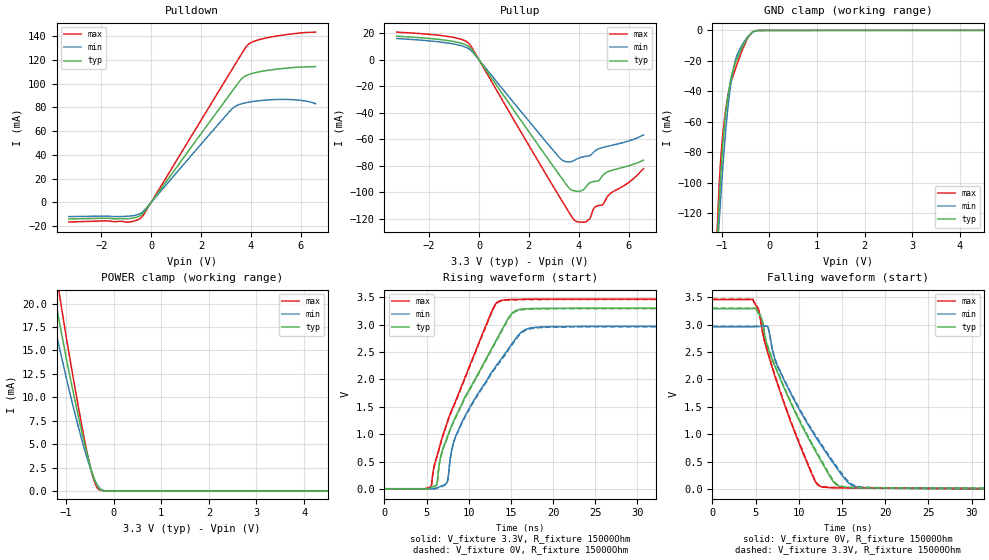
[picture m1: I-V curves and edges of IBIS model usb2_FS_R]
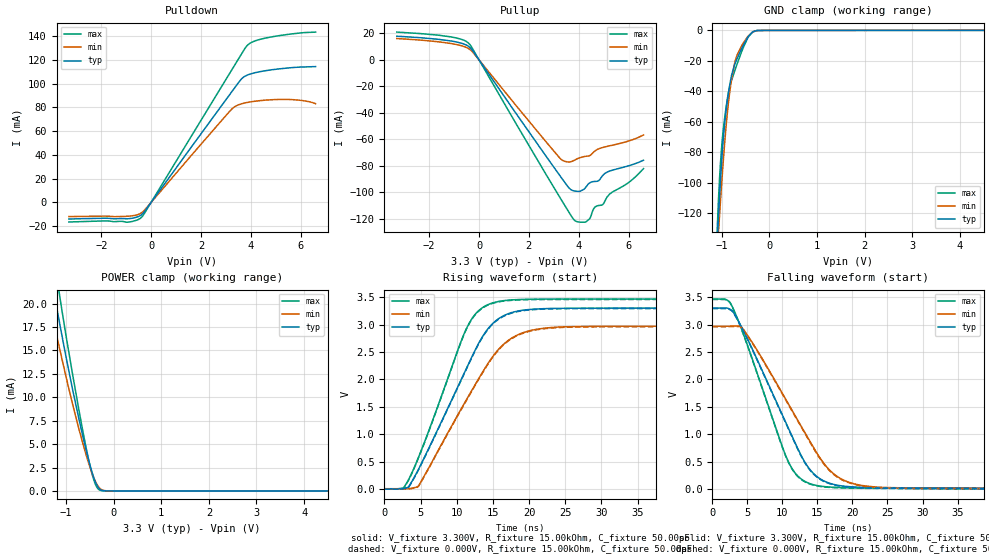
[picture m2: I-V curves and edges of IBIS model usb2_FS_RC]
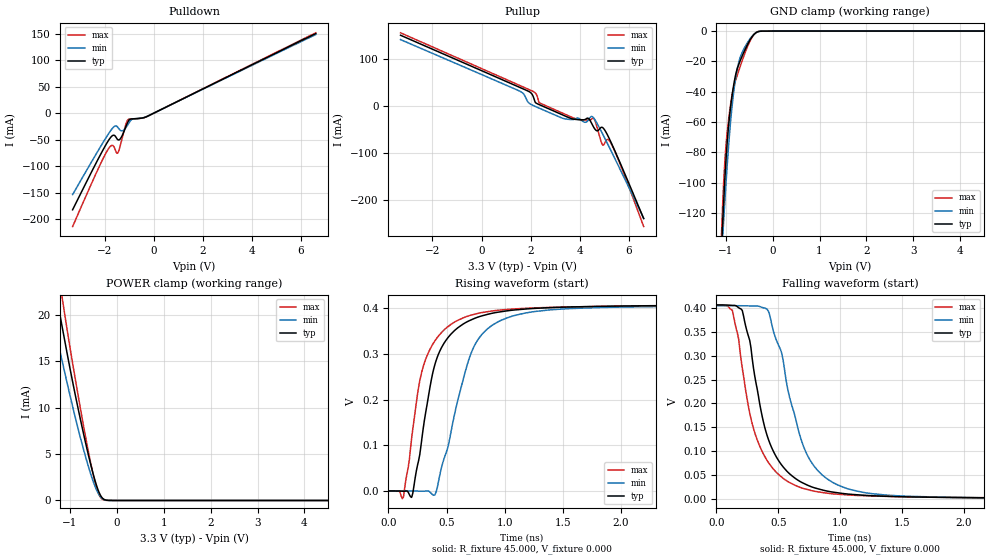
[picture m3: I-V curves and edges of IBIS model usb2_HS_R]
| Texas Instruments Incorporated
| Four-Port USB 2.0 Hub
| Marketing part#   Voltage Range   Package-type   Temperature
| TUSB4041PAP   2.97V - 3.465V   64-Pin PAP   -40 to 85 C
[IBIS Ver]   4.1
[File name]   tusb4041IPAP.ibs
[File Rev]   1.0
[Date]   05/22/2014
[Source]   Model built from TISPICE simulations at:
   Texas Instruments Incorporated.
   Analog-eLab, HPA
   12500 TI Blvd
   Dallas, TX -75243
[Notes]   Rev 1.0: 09/08/2017
   - Model based on v1.0 IBIS model for TUSB8041q1 dated 02/28/2014
[Disclaimer] This product is designed as an aid for customers of Texas Instruments.
   No warranties, either expressed or implied, with respect to this third
   party software (if any) or with respect to its fitness for any
   particular purpose is claimed by Texas Instruments or the author. The
   software (if any) is provided solely on an "as is" basis. The entire
   risk as to its quality and performance is with the customer
[Copyright]   (C)Copyright 2014 Texas Instruments Incorporated.
   All rights reserved.
|   TUSB8041
[Component]   TUSB4041
[Manufacturer]  Texas Instruments Incorporated
[Package]   |64-pin PAP
|   typ   min   max
R_pkg   0.2389   0.0142   0.3346
L_pkg   2.3741nH   1.4298nH   2.8522nH
C_pkg   0.8499pF   0.7143pF   1.0609pF
[PIN]   signal_name   model_name   R_pin   L_pin   C_pin
1   PWRCTL3/BATEN3   BC3340DSHYPBFZP18PD   NA   NA   NA
2   VDD33   POWER   NA   NA   NA
3   PWRCTL2/BATEN2   BC3340DSHYPBFZP18PD   NA   NA   NA
4   PWRCTL1/BATEN1   BC3340DSHYPBFZP18PD   NA   NA   NA
5   SDA/SMBDAT   BC3340DSHYPBFZP18PD   NA   NA   NA
6   SCL/SMBCLK   BC3340DSHYPBFZP18PD   NA   NA   NA
7   SMBUSZ   BC3340DSHYPBFZP18PU   NA   NA   NA
8   FULLPWRMGMTz/SMBA1   BC3340DSHYPBFZP18PD   NA   NA   NA
9   POWCTL_POL   BC3340DSHYPBFZP18PU   NA   NA   NA
10   GANGED/SMBAS2/HS_UP   BC3340DSHYPBFZP18PD   NA   NA   NA
11   OVERCUR4Z   IC33SHYPBFZP18PU   NA   NA   NA
12   OVERCUR3Z   IC33SHYPBFZP18PU   NA   NA   NA
13   AUTOENZ/HS_SUSPEND   BC3340DSHYPBFZP18PU   NA   NA   NA
14   OVERCUR1Z   IC33SHYPBFZP18PU   NA   NA   NA
15   OVERCUR2Z   IC33SHYPBFZP18PU   NA   NA   NA
16   USB_VBUS   IC33SHYPBFZP18   NA   NA   NA
17   TEST   IC33SHYPBFZP18PD   NA   NA   NA
18   GRSTZ   IC33SHYPBFZP18PU   NA   NA   NA
19   VDD   POWER   NA   NA   NA
20   VDD33   POWER   NA   NA   NA
21   USB_DP_UP   usb2   NA   NA   NA
22   USB_DM_UP   usb2   NA   NA   NA
23   RSVD   NC   NA   NA   NA
24   RSVD   NC   NA   NA   NA
25   VDD   POWER   NA   NA   NA
26   RSVD   NC   NA   NA   NA
27   RSVD   NC   NA   NA   NA
28   NC   NC   NA   NA   NA
29   XO   NC   NA   NA   NA
30   XI   NC   NA   NA   NA
31   VDD33   POWER   NA   NA   NA
32   USB_R1   NC   NA   NA   NA
33   USB_DP_DN1   usb2   NA   NA   NA
34   USB_DM_DN1   usb2   NA   NA   NA
35   RSVD   NC   NA   NA   NA
36   RSVD   NC   NA   NA   NA
37   VDD   POWER   NA   NA   NA
38   RSVD   NC   NA   NA   NA
39   RSVD   NC   NA   NA   NA
40   NC   NC   NA   NA   NA
41   USB_DP_DN2   usb2   NA   NA   NA
42   USB_DM_DN2   usb2   NA   NA   NA
43   RSVD   NC   NA   NA   NA
44   RSVD   NC   NA   NA   NA
45   VDD   POWER   NA   NA   NA
46   RSVD   NC   NA   NA   NA
47   RSVD   NC   NA   NA   NA
48   VDD33   POWER   NA   NA   NA
49   USB_DP_DN3   usb2   NA   NA   NA
50   USB_DM_DN3   usb2   NA   NA   NA
51   RSVD   NC   NA   NA   NA
52   RSVD   NC   NA   NA   NA
53   VDD   POWER   NA   NA   NA
54   RSVD   NC   NA   NA   NA
55   RSVD   NC   NA   NA   NA
56   USB_DP_DN4   usb2   NA   NA   NA
57   USB_DM_DN4   usb2   NA   NA   NA
58   RSVD   NC   NA   NA   NA
59   RSVD   NC   NA   NA   NA
60   VDD   POWER   NA   NA   NA
61   RSVD   NC   NA   NA   NA
62   RSVD   NC   NA   NA   NA
63   VDD   POWER   NA   NA   NA
64   PWRCTL4/BATEN4   BC3340DSHYPBFZP18PD   NA   NA   NA
[Diff_pin]   inv_pin   vdiff   tdelay_typ   tdelay_min   tdelay_max
21   22   NA   NA   NA   NA
33   34   NA   NA   NA   NA
41   42   NA   NA   NA   NA
49   50   NA   NA   NA   NA
56   57   NA   NA   NA   NA
[Model Selector] usb2
usb2_HS_R   USB 2.0 High Speed mode, for DP/DM pin 240MHz
usb2_HS_RC   USB 2.0 High Speed mode, for DP/DM pin 240MHz, with Cfixture
usb2_FS_R   USB 2.0 Fast Speed mode, for DP/DM pin 6MHz
usb2_FS_RC   USB 2.0 Fast Speed mode, for DP/DM pin 6MHz, with Cfixture
usb2_LS_RC   USB 2.0 Low  Speed mode, for DP/DM pin 750kHz, with Cfixture
usb2_LS_R   USB 2.0 Low  Speed mode, for DP/DM pin 750kHz
[Model Selector] BC3340DSHYPBFZP18
HYPBFZP18_PI_5P_3P3 BUFFER WITHOUT PULLUP/PULLDOWN & 5% VDDS TOLERANCE
HYPBFZP18_PI_10P_3P3 BUFFER WITHOUT PULLUP/PULLDOWN & 10% VDDS TOLERANCE
[Model Selector] BC3340DSHYPBFZP18PU
FZP18_PU_PI_5P_3P3 BUFFER WITH WEAK PULLUP & 5% VDDS TOLERANCE
FZP18_PU_PI_10P_3P3 BUFFER WITH WEAK PULLUP & 10% VDDS TOLERANCE
[Model Selector] BC3340DSHYPBFZP18PD
FZP18_PD_PI_5P_3P3 BUFFER WITH WEAK PULLDOWN & 5% VDDS TOLERANCE
FZP18_PD_PI_10P_3P3 BUFFER WITH WEAK PULLDOWN & 10% VDDS TOLERANCE
[Model Selector] IC33SHYPBFZP18
C33SHYPBFZP18_10P BUFFER WITHOUT PULLUP/PULLDOWN & 10% VDDS TOLERANCE
C33SHYPBFZP18_5P  BUFFER WITHOUT PULLUP/PULLDOWN & 5% VDDS TOLERANCE
[Model Selector] IC33SHYPBFZP18PD
YPBFZP18_PD_5P BUFFER with WEAK PULLDOWN & 5% VDDS TOLERANCE
YPBFZP18_PD_10P BUFFER with WEAK PULLDOWN & 5% VDDS TOLERANCE
[Model Selector] IC33SHYPBFZP18PU
PBFZP18_PU_5P BUFFER with WEAK PULLUP & 5% VDDS TOLERANCE
PBFZP18_PU_10P BUFFER with WEAK PULLUP & 10% VDDS TOLERANCE
| Models and submodels in the file (18): usb2_FS_R (I/O), usb2_FS_RC (I/O), usb2_HS_R (I/O), usb2_HS_RC (I/O), usb2_LS_R (I/O), usb2_LS_RC (I/O), HYPBFZP18_PI_5P_3P3 (I/O), HYPBFZP18_PI_10P_3P3 (I/O), FZP18_PU_PI_5P_3P3 (I/O), FZP18_PU_PI_10P_3P3 (I/O), FZP18_PD_PI_5P_3P3 (I/O), FZP18_PD_PI_10P_3P3 (I/O), YPBFZP18_PD_10P (Input), PBFZP18_PU_10P (Input), C33SHYPBFZP18_10P (Input), YPBFZP18_PD_5P (Input), PBFZP18_PU_5P (Input), C33SHYPBFZP18_5P (Input)
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|   USB 2.0 Fast Speed mode, for DP pin 6MHz
[Model]   usb2_FS_R
Model_type   I/O
Polarity   Non-Inverting
Enable   Active-High
Vmeas = 1.54
Vref = 0
Rref = 15000
Cref = 50pF
Vinl = 0.8V
Vinh = 2.0V
|   typ   min   max
|   (nom PVT)   (Fast PVT)   (slow PVT)
C_comp   9.0376pF   8.9385pF   9.1512pF
[Voltage Range]   3.3   2.97   3.465
[Temperature Range]   27   105   -40
[Pullup Reference]   3.3   2.97   3.465
[Pulldown Reference]   -0   -0   -0
[Power Clamp Reference]   3.3   2.97   3.465
[GND Clamp Reference]   -0   -0   -0
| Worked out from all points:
|   slope of the pulldown table from 0 to 0.495 V, typ, clamps not added: 34.6 ohm
|   slope of the pullup table from 0 to 0.495 V, typ, clamps not added: 36.8 ohm
|   GND clamp passes 1 mA (typ) near -0.35 V on its own axis
|   POWER clamp passes 1 mA (typ) near -0.39 V on its own axis
|   falling waveform, V_fixture 0V, R_fixture 15000Ohm: 20-80 % time 5.73ns typ, 6.23ns min, 4.47ns max; typ from 3.29 V to 0 V
|   rising waveform, V_fixture 3.3V, R_fixture 15000Ohm: 20-80 % time 6.21ns typ, 6.02ns min, 5.07ns max; typ from 0.008 V to 3.3 V
|   rising waveform, V_fixture 0V, R_fixture 15000Ohm: 20-80 % time 6.24ns typ, 6.08ns min, 5.09ns max; typ from 0 V to 3.29 V
|   falling waveform, V_fixture 3.3V, R_fixture 15000Ohm: 20-80 % time 5.77ns typ, 6.3ns min, 4.5ns max; typ from 3.3 V to 0.008 V
[Pulldown]
|   Voltage   I(typ)   I(min)   I(max)
-3.3V     -13.97mA   -11.94mA   -16.5mA
-1.865V   -13.31mA   -11.55mA   -15.58mA
-948.8mV  -13.78mA   -11.64mA   -16.64mA
-429mV    -11.05mA   -9.328mA   -13.36mA
-255.8mV  -7.37mA    -6.247mA   -8.827mA
3.234V    93.1mA     78.54mA    111.5mA
3.61V     103.6mA    82.92mA    124.4mA
3.858V    107.2mA    84.17mA    132.2mA
4.15V     109.1mA    85.16mA    135.8mA
4.714V    111.3mA    86.32mA    138.9mA
5.798V    113.7mA    86.37mA    142.3mA
6.6V      114.4mA    83.14mA    143.4mA
[GND Clamp]
|   Voltage   I(typ)   I(min)   I(max)
-3.3V     -2.986A    -2.594A    -3.408A
-1.102V   -142.8mA   -148.5mA   -133.6mA
-1.068V   -120.4mA   -130.9mA   -108.6mA
-1.053V   -111.5mA   -123.5mA   -99.43mA
-1.028V   -97.72mA   -111.6mA   -86.34mA
-948.8mV  -63.66mA   -76.9mA    -59.29mA
-874.5mV  -43.76mA   -51.14mA   -43.02mA
-795.3mV  -29.32mA   -31.84mA   -32.77mA
-676.5mV  -18.29mA   -15.93mA   -21.75mA
-458.7mV  -4.679mA   -4.168mA   -5.163mA
-349.8mV  -954.6uA   -1.019mA   -868.7uA
6.6V      27.44uA    21.44uA    34.47uA
[Pullup]
|   Voltage   I(typ)   I(min)   I(max)
-3.3V     17.86mA    16.11mA    20.95mA
-1.162V   14.34mA    12.44mA    17.42mA
-374.6mV  9.504mA    7.922mA    11.72mA
3.224V    -86.72mA   -73.66mA   -103.1mA
3.625V    -96.87mA   -77.02mA   -115.4mA
3.863V    -98.94mA   -75.34mA   -121.4mA
4.303V    -95.54mA   -72.68mA   -122mA
4.452V    -92.62mA   -72.08mA   -119.5mA
4.655V    -91.65mA   -68.64mA   -111mA
4.962V    -87.23mA   -66.09mA   -109.1mA
5.14V     -84.63mA   -65.26mA   -103.4mA
6.6V      -75.66mA   -56.61mA   -82.01mA
[POWER Clamp]
|   Voltage   I(typ)   I(min)   I(max)
-3.3V     96.11mA    80.39mA    114.3mA
-1.409V   25.5mA     21.48mA    30.05mA
-1.315V   22.86mA    19.29mA    26.86mA
-1.246V   20.93mA    17.7mA     24.52mA
-1.127V   17.68mA    15mA       20.59mA
-854.7mV  10.64mA    9.089mA    12.22mA
-567.6mV  4.132mA    3.664mA    4.338mA
-419.1mV  1.439mA    1.425mA    1.205mA
-359.7mV  684.8uA    768.2uA    455.6uA
-290.4mV  187uA      273.4uA    86.97uA
0V        0A         0A         0A
6.6V      0A         0A         0A
[Ramp]
R_load = 15000
|   typ   min   max
dV/dt_r   1.97481/6.20846e-009   1.77621/6.02152e-009   2.07437/5.07374e-009
dV/dt_f   1.97455/5.7255e-009   1.77598/6.2317e-009   2.07413/4.47102e-009
[Falling Waveform]
V_fixture = 0V
V_fixture_min = 0V
V_fixture_max = 0V
R_fixture = 15000Ohm
C_fixture = 0F
|   Time   V(typ)   V(min)   V(max)
0s        3.291V     2.961V     3.457V
4.7ns     3.293V     2.961V     3.458V
5.7ns     3.108V     2.967V     2.957V
6.4ns     2.601V     2.967V     2.494V
7.5ns     2.143V     2.254V     1.936V
11.4ns    846.1mV    1.091V     316.1mV
12.6ns    506.4mV    796.2mV    44.4mV
14.4ns    75.51mV    384.1mV    24.24mV
17.5ns    21.5mV     25.98mV    19.1mV
84.9ns    94.35uV    653.8uV    37.35uV
[Rising Waveform]
|Vcc
V_fixture = 3.3V
V_fixture_min = 2.97V
V_fixture_max = 3.465V
R_fixture = 15000Ohm
C_fixture = 0F
|   Time   V(typ)   V(min)   V(max)
0s        7.658mV    8.716mV    6.679mV
5.5ns     34.03mV    9.217mV    46.24mV
6.2ns     85.76mV    22.01mV    590.8mV
6.6ns     542.7mV    47.18mV    807.5mV
7.4ns     926.5mV    115.1mV    1.193V
8.6ns     1.371V     1.019V     1.668V
13.8ns    2.867V     2.361V     3.438V
15.3ns    3.227V     2.686V     3.457V
18.1ns    3.293V     2.951V     3.462V
84.9ns    3.299V     2.969V     3.464V
[Rising Waveform]
V_fixture = 0V
V_fixture_min = 0V
V_fixture_max = 0V
R_fixture = 15000Ohm
C_fixture = 0F
|   Time   V(typ)   V(min)   V(max)
0s        100.2uV    720.6uV    39.4uV
5.5ns     26.33mV    1.222mV    39.41mV
6.2ns     77.72mV    13.9mV     579.6mV
6.6ns     530.5mV    39.01mV    795.4mV
7.4ns     911.9mV    106.6mV    1.179V
8.6ns     1.353V     1.003V     1.653V
13.8ns    2.848V     2.339V     3.429V
15.5ns    3.233V     2.707V     3.45V
18.3ns    3.285V     2.942V     3.455V
84.9ns    3.291V     2.961V     3.457V
[Falling Waveform]
|Gnd
V_fixture = 3.3V
V_fixture_min = 2.97V
V_fixture_max = 3.465V
R_fixture = 15000Ohm
C_fixture = 0F
|   Time   V(typ)   V(min)   V(max)
0s        3.299V     2.969V     3.464V
4.7ns     3.301V     2.97V      3.465V
5.7ns     3.117V     2.975V     2.966V
6.4ns     2.614V     2.976V     2.506V
7.5ns     2.159V     2.27V      1.952V
11.5ns    841mV      1.091V     299.3mV
12.7ns    502.5mV    798.8mV    49.57mV
14.4ns    91.03mV    411.2mV    31.27mV
17.6ns    29.38mV    35.57mV    25.66mV
84.9ns    7.652mV    8.648mV    6.677mV
|   USB 2.0 Fast Speed mode, for DM pin 6MHz
[Model]   usb2_FS_RC
Model_type   I/O
Polarity   Non-Inverting
Enable   Active-High
Vmeas = 1.54
Vref = 0
Rref = 15000
Cref = 50pF
Vinl = 0.8V
Vinh = 2.0V
|   typ   min   max
|   (nom PVT)   (Fast PVT)   (slow PVT)
C_comp   9.0376pF   8.9385pF   9.1512pF
[Voltage Range]   3.3   2.97   3.465
[Temperature Range]   27   105   -40
[Pullup Reference]   3.3   2.97   3.465
[Pulldown Reference]   -0   -0   -0
[Power Clamp Reference]   3.3   2.97   3.465
[GND Clamp Reference]   -0   -0   -0
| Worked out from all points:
|   slope of the pulldown table from 0 to 0.495 V, typ, clamps not added: 34.6 ohm
|   slope of the pullup table from 0 to 0.495 V, typ, clamps not added: 36.8 ohm
|   GND clamp passes 1 mA (typ) near -0.35 V on its own axis
|   POWER clamp passes 1 mA (typ) near -0.39 V on its own axis
|   falling waveform, V_fixture 3.300V, R_fixture 15.00kOhm, C_fixture 50.00pF: 20-80 % time 7.09ns typ, 8.08ns min, 5.62ns max; typ from 3.3 V to 0.008 V
|   rising waveform, V_fixture 3.300V, R_fixture 15.00kOhm, C_fixture 50.00pF: 20-80 % time 7.12ns typ, 7.76ns min, 5.77ns max; typ from 0.008 V to 3.3 V
|   rising waveform, V_fixture 0.000V, R_fixture 15.00kOhm, C_fixture 50.00pF: 20-80 % time 7.12ns typ, 7.77ns min, 5.77ns max; typ from 0 V to 3.29 V
|   falling waveform, V_fixture 0.000V, R_fixture 15.00kOhm, C_fixture 50.00pF: 20-80 % time 7.08ns typ, 8.07ns min, 5.61ns max; typ from 3.29 V to 0 V
[Pulldown]
|   Voltage   I(typ)   I(min)   I(max)
-3.3V     -13.97mA   -11.94mA   -16.5mA
-1.865V   -13.31mA   -11.55mA   -15.58mA
-948.8mV  -13.78mA   -11.64mA   -16.64mA
-429mV    -11.05mA   -9.328mA   -13.36mA
-255.8mV  -7.37mA    -6.247mA   -8.827mA
3.234V    93.1mA     78.54mA    111.5mA
3.61V     103.6mA    82.92mA    124.4mA
3.858V    107.2mA    84.17mA    132.2mA
4.15V     109.1mA    85.16mA    135.8mA
4.714V    111.3mA    86.32mA    138.9mA
5.798V    113.7mA    86.37mA    142.3mA
6.6V      114.4mA    83.14mA    143.4mA
[GND Clamp]
|   Voltage   I(typ)   I(min)   I(max)
-3.3V     -2.986A    -2.594A    -3.408A
-1.102V   -142.8mA   -148.5mA   -133.6mA
-1.068V   -120.4mA   -130.9mA   -108.6mA
-1.053V   -111.5mA   -123.5mA   -99.43mA
-1.028V   -97.72mA   -111.6mA   -86.34mA
-948.8mV  -63.66mA   -76.9mA    -59.29mA
-874.5mV  -43.76mA   -51.14mA   -43.02mA
-795.3mV  -29.32mA   -31.84mA   -32.77mA
-676.5mV  -18.29mA   -15.93mA   -21.75mA
-458.7mV  -4.679mA   -4.168mA   -5.163mA
-349.8mV  -954.6uA   -1.019mA   -868.7uA
6.6V      27.44uA    21.44uA    34.47uA
[Pullup]
|   Voltage   I(typ)   I(min)   I(max)
-3.3V     17.86mA    16.11mA    20.95mA
-1.162V   14.34mA    12.44mA    17.42mA
-374.6mV  9.504mA    7.922mA    11.72mA
3.224V    -86.72mA   -73.66mA   -103.1mA
3.625V    -96.87mA   -77.02mA   -115.4mA
3.863V    -98.94mA   -75.34mA   -121.4mA
4.303V    -95.54mA   -72.68mA   -122mA
4.452V    -92.62mA   -72.08mA   -119.5mA
4.655V    -91.65mA   -68.64mA   -111mA
4.962V    -87.23mA   -66.09mA   -109.1mA
5.14V     -84.63mA   -65.26mA   -103.4mA
6.6V      -75.66mA   -56.61mA   -82.01mA
[POWER Clamp]
|   Voltage   I(typ)   I(min)   I(max)
-3.3V     96.11mA    80.39mA    114.3mA
-1.409V   25.5mA     21.48mA    30.05mA
-1.315V   22.86mA    19.29mA    26.86mA
-1.246V   20.93mA    17.7mA     24.52mA
-1.127V   17.68mA    15mA       20.59mA
-854.7mV  10.64mA    9.089mA    12.22mA
-567.6mV  4.132mA    3.664mA    4.338mA
-419.1mV  1.439mA    1.425mA    1.205mA
-359.7mV  684.8uA    768.2uA    455.6uA
-290.4mV  187uA      273.4uA    86.97uA
0V        0A         0A         0A
6.6V      0A         0A         0A
[Ramp]
R_load = 15.00kOhm
|   typ   min   max
dV/dt_r   1.975V/7.118ns   1.776V/7.768ns   2.074V/5.764ns
dV/dt_f   1.975V/7.089ns   1.777V/8.081ns   2.074V/5.614ns
[Falling Waveform]
V_fixture = 3.300V
V_fixture_min = 2.970V
V_fixture_max = 3.465V
R_fixture = 15.00kOhm
C_fixture = 50.00pF
|   Time   V(typ)   V(min)   V(max)
0s        3.299V     2.969V     3.464V
2.4ns     3.286V     2.97V      3.419V
4.2ns     2.947V     2.947V     2.907V
10.69ns   1.157V     1.59V      545mV
12.14ns   753.6mV    1.267V     246.5mV
14.07ns   335.9mV    840.6mV    94.42mV
15.85ns   154.3mV    481.3mV    48.71mV
17.64ns   77.37mV    248.2mV    32.68mV
22.25ns   29.92mV    52.16mV    21.45mV
83.29ns   7.582mV    8.019mV    6.667mV
[Rising Waveform]
V_fixture = 3.300V
V_fixture_min = 2.970V
V_fixture_max = 3.465V
R_fixture = 15.00kOhm
C_fixture = 50.00pF
|   Time   V(typ)   V(min)   V(max)
0s        7.582mV    8.019mV    6.667mV
2.63ns    14.86mV    8.107mV    23.09mV
3.35ns    42.86mV    10.65mV    176.9mV
4.68ns    354.6mV    57.1mV     571.4mV
11.34ns   2.202V     1.63V      2.927V
12.88ns   2.621V     1.981V     3.234V
14.9ns    3.01V      2.403V     3.391V
18.36ns   3.243V     2.808V     3.454V
23.8ns    3.294V     2.952V     3.463V
83.29ns   3.299V     2.969V     3.464V
[Rising Waveform]
V_fixture = 0.000V
V_fixture_min = 0.000V
V_fixture_max = 0.000V
R_fixture = 15.00kOhm
C_fixture = 50.00pF
|   Time   V(typ)   V(min)   V(max)
0s        3.197uV    8.923uV    4.349uV
2.63ns    7.278mV    96.94uV    16.39mV
3.36ns    36.84mV    2.771mV    171.8mV
4.68ns    345.4mV    48.95mV    562.8mV
11.35ns   2.193V     1.621V     2.921V
12.89ns   2.613V     1.97V      3.227V
14.91ns   3.001V     2.393V     3.384V
18.18ns   3.229V     2.786V     3.446V
23.01ns   3.284V     2.936V     3.456V
83.29ns   3.291V     2.961V     3.457V
[Falling Waveform]
V_fixture = 0.000V
V_fixture_min = 0.000V
V_fixture_max = 0.000V
R_fixture = 15.00kOhm
C_fixture = 50.00pF
|   Time   V(typ)   V(min)   V(max)
0s        3.291V     2.961V     3.457V
2.4ns     3.278V     2.961V     3.412V
4.2ns     2.937V     2.938V     2.898V
10.67ns   1.15V      1.581V     540.7mV
12.12ns   746.6mV    1.258V     240.7mV
14.05ns   328.3mV    831mV      87.96mV
15.83ns   146.5mV    471.7mV    42.08mV
17.61ns   69.9mV     239.9mV    26.07mV
22.23ns   22.29mV    43.83mV    14.8mV
83.29ns   3.197uV    8.923uV    4.349uV
|   USB 2.0 High Speed mode, for DP pin 240MHz (Internal Termination ON)
[Model]   usb2_HS_R
Model_type   I/O
Polarity   Non-Inverting
Enable   Active-High
Vmeas = 202mV
Vref = 0
Rref = 45
Cref =1pF
Vinl = 150mV
Vinh = 360mV
|   typ   min   max
|EXCEPTION   (nom PVT)   (Slow PVT) (Fast PVT)
C_comp   6.3538pF   6.1002pF   6.4829pF
|5.8941pF   5.4228pF   6.1646pF
[Voltage Range]   3.3   2.97   3.465
[Temperature Range]   27   105   -40
[Pullup Reference]   3.3   2.97   3.465
[Pulldown Reference]   0   0   0
[Power Clamp Reference]   3.3   2.97   3.465
[GND Clamp Reference]   0   0   0
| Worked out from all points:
|   slope of the pulldown table from 0 to 0.495 V, typ, clamps not added: 43.6 ohm
|   slope of the pullup table from 0 to 0.495 V, typ, clamps not added: 43.7 ohm
|   GND clamp passes 1 mA (typ) near -0.35 V on its own axis
|   POWER clamp passes 1 mA (typ) near -0.39 V on its own axis
|   rising waveform, R_fixture 45.000, V_fixture 0.000: 20-80 % time 214ps typ, 261ps min, 207ps max; typ from 0 V to 0.407 V
|   falling waveform, R_fixture 45.000, V_fixture 0.000: 20-80 % time 225ps typ, 258ps min, 223ps max; typ from 0.407 V to 0 V
[Pulldown]
|   Voltage   I(typ)   I(min)   I(max)
-3.3V     -182.7mA   -154mA     -214.5mA
-2.109V   -73.47mA   -59.12mA   -90.55mA
-1.836V   -51.34mA   -38.81mA   -67.06mA
-1.687V   -42.74mA   -29.04mA   -60.76mA
-1.588V   -42.26mA   -24.56mA   -66.11mA
-1.464V   -49.94mA   -26.46mA   -75.27mA
-1.265V   -40.67mA   -33.14mA   -44.1mA
-1.141V   -26.63mA   -28.06mA   -22.45mA
-1.042V   -16mA      -21.02mA   -12.18mA
-868.4mV  -10.68mA   -11.28mA   -10.85mA
-297.7mV  -6.74mA    -6.624mA   -6.826mA
6.6V      150.7mA    148.8mA    152.1mA
[GND Clamp]
|   Voltage   I(typ)   I(min)   I(max)
-3.3V     -3.521A    -2.996A    -4.111A
-1.092V   -145.9mA   -151.2mA   -136.4mA
-1.067V   -128.4mA   -137.7mA   -116.4mA
-1.042V   -112.2mA   -124.7mA   -99.36mA
-1.017V   -97.56mA   -112.1mA   -85.68mA
-967.7mV  -73.5mA    -88.57mA   -66.63mA
-893.2mV  -49.51mA   -59.02mA   -47.86mA
-818.8mV  -33.69mA   -37.74mA   -35.76mA
-669.9mV  -17.99mA   -15.57mA   -21.42mA
-471.4mV  -5.326mA   -4.698mA   -5.944mA
-322.6mV  -523.8uA   -615.4uA   -432uA
6.6V      27.34uA    21.38uA    34.43uA
[Pullup]
|   Voltage   I(typ)   I(min)   I(max)
-3.3V     150.7mA    141.5mA    155.9mA
1.588V    39.24mA    31.21mA    43.36mA
2.084V    22.84mA    2.078mA    31.83mA
2.357V    3.277mA    -4.287mA   7.257mA
3.25V     -17.25mA   -24.5mA    -13.49mA
4.342V    -25.52mA   -29.54mA   -29.28mA
4.565V    -44.49mA   -24.78mA   -25.96mA
4.714V    -52.12mA   -37.54mA   -46.83mA
4.913V    -44.86mA   -57.23mA   -80.87mA
5.086V    -57mA      -75.14mA   -71.32mA
5.434V    -95.43mA   -111.8mA   -96.58mA
6.6V      -238.4mA   -237.7mA   -255.4mA
[POWER Clamp]
|   Voltage   I(typ)   I(min)   I(max)
-3.3V     96.73mA    79.76mA    115.2mA
-1.439V   26.41mA    21.36mA    31.18mA
-1.265V   21.53mA    17.34mA    25.27mA
-1.241V   20.85mA    16.77mA    24.43mA
-1.141V   18.11mA    14.53mA    21.12mA
-843.6mV  10.39mA    8.125mA    11.91mA
-570.7mV  4.197mA    3.107mA    4.415mA
-421.8mV  1.476mA    1.033mA    1.243mA
-372.2mV  816.7uA    565.7uA    573.1uA
-297.7mV  217.2uA    160.3uA    102.4uA
0V        0A         0A         0A
6.6V      0A         0A         0A
[Ramp]
R_load = 45
|   typ   min   max
dV/dt_r   0.241436/2.13719e-10   0.240166/2.60796e-10   0.241677/2.07061e-10
dV/dt_f   0.241444/2.2514e-10   0.240152/2.57832e-10   0.241591/2.23371e-10
[Rising Waveform]
R_fixture = 45.000
V_fixture = 0.000
V_fixture_min = 0.000
V_fixture_max = 0.000
|  time   V(typ)   V(min)   V(max)
0s        11.24uV    5.401uV    22.98uV
130ps     -771.8uV   -133.3uV   -13.14mV
200ps     -14.17mV   -290.1uV   114.9mV
280ps     98.17mV    -662uV     252.8mV
400ps     276.5mV    -8.747mV   328.3mV
600ps     357.5mV    201.2mV    373.6mV
700ps     372.9mV    293.4mV    383.8mV
780ps     381.2mV    334.5mV    389mV
1.08ns    395.8mV    383.6mV    398.2mV
3.4ns     407mV      405.3mV    406.8mV
[Falling Waveform]
R_fixture = 45.000
V_fixture = 0.000
V_fixture_min = 0.000
V_fixture_max = 0.000
|  time   V(typ)   V(min)   V(max)
0s        407mV      405.3mV    406.8mV
130ps     406mV      405.4mV    395.7mV
210ps     395.4mV    405.3mV    274.2mV
300ps     275.3mV    404.8mV    148mV
420ps     125.3mV    394.3mV    76.43mV
530ps     70.04mV    303.9mV    44.94mV
640ps     42.29mV    169.1mV    27.77mV
790ps     23.09mV    68.43mV    15.83mV
1.08ns    9.333mV    19.46mV    7.581mV
3.4ns     11.24uV    5.401uV    22.98uV
